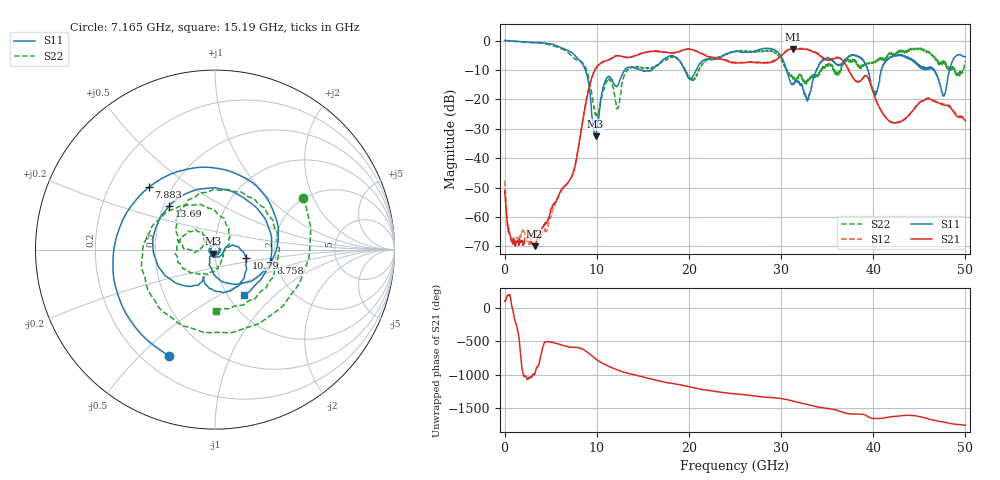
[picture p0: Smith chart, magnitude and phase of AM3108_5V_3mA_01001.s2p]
# Hz S DB R 50.0
!freq dBS11 angS11 dBS21 angS21 dBS12 angS12 dBS22 angS22
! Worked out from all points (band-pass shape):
!   1601 points, 10 MHz to 50 GHz, reference 50 ohm
!   highest |S21| = -2.83 dB at 31.28 GHz (marker M1); lowest = -69.9 dB at 3.259 GHz (marker M2)
!   |S21| within 3 dB of the highest: 11.75 GHz to 22.64 GHz (10.89 GHz wide, 63.3 % of centre); 29.79 GHz to 34.46 GHz (4.667 GHz wide, 14.5 % of centre)
!   lowest |S11| = -32.5 dB at 9.883 GHz (marker M3), VSWR 1.05, Z = 49.1 - j2.14 ohm
!   |S11| at or under -10 dB: 8.771 GHz to 13.04 GHz (4.272 GHz wide, 39.2 % of centre); 30.61 GHz to 33.84 GHz (3.235 GHz wide, 10 % of centre); 46.63 GHz to 48.28 GHz (1.652 GHz wide, 3.48 % of centre)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
!   |S22| runs from -26.0 to 0.0 dB; largest |S21 - S12| = 0.024
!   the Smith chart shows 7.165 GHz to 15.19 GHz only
!   S11 on the Smith chart (normalised r, x): 7.165 GHz: 0.30, -0.61; 7.883 GHz: 0.37, +0.35; 8.758 GHz: 1.87, -0.30; 10.79 GHz: 1.41, -0.13; 13.69 GHz: 0.54, +0.29; 15.19 GHz: 1.19, -0.66
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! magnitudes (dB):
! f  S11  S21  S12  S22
! 10 MHz  0.0  -51.1  -47.6  0.0
! 822.3 MHz  -0.1  -68.3  -68.7  -0.2
! 3.259 GHz  -0.7  -69.9  -65.6  -0.8
! 7.165 GHz  -3.8  -47.0  -46.9  -4.9
! 7.883 GHz  -5.9  -38.9  -38.7  -6.5
! 8.352 GHz  -7.5  -29.9  -29.8  -7.2
! 8.758 GHz  -9.9  -22.3  -22.2  -9.0
! 9.883 GHz  -32.5  -9.6  -9.6  -24.8
! 10.79 GHz  -14.9  -7.2  -7.0  -16.7
! 12.26 GHz  -15.3  -5.2  -5.1  -23.3
! 13.69 GHz  -9.1  -5.7  -5.6  -9.4
! 15.19 GHz  -10.5  -4.1  -4.0  -9.4
! 16.69 GHz  -8.2  -3.8  -3.5  -8.3
! 25 GHz  -3.7  -7.6  -7.5  -3.8
! 29.38 GHz  -3.3  -6.8  -6.6  -4.1
! 31.28 GHz  -15.0  -2.8  -2.7  -13.1
! 33.35 GHz  -15.6  -3.7  -3.4  -12.7
! 37.88 GHz  -4.8  -13.0  -13.0  -6.5
! 40.22 GHz  -18.7  -19.7  -19.6  -7.6
! 41.69 GHz  -6.1  -27.2  -27.2  -5.2
! 47.66 GHz  -19.0  -21.9  -21.6  -7.7
! 50 GHz  -5.5  -27.2  -26.7  -6.9
